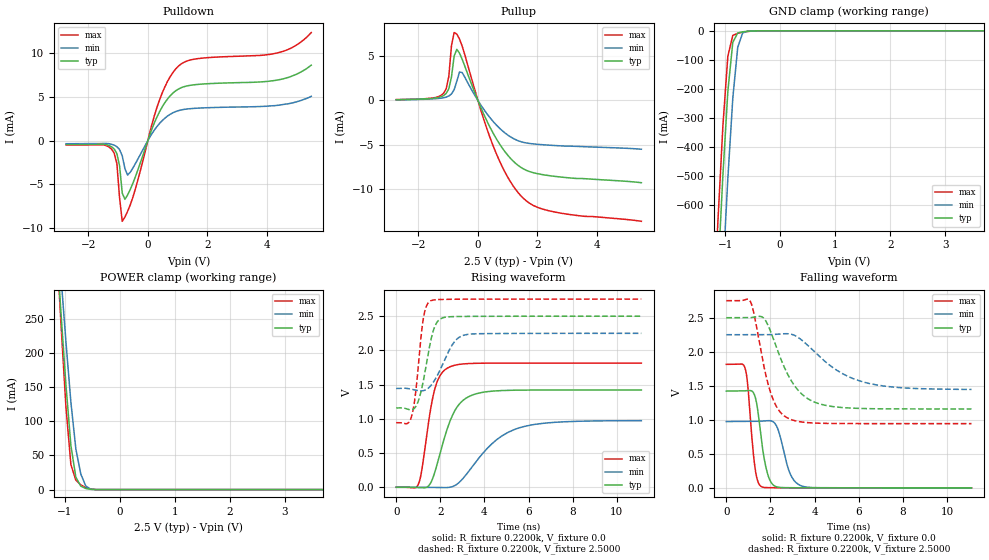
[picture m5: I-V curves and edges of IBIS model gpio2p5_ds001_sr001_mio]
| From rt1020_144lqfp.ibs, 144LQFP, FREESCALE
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[Model] gpio2p5_ds001_sr001_mio
|   Model gpio2p5_ds001_sr001_mio
| This model was characterised for following simulation conditions:
| External (pad) voltage:
|   - Typ: 2.5V,   - Min: 2.25V,   - Max: 2.75V
| Library cells for typ/min/max conditions are connected as defined below:
|  pad - External Pad
|  ipp_do - Core Input
|  ipp_obe - Output Buffer Enable
|  esd_boost - ovdd
|  ipp_dse0 - vddi
|  ipp_dse1 - vssi
|  ipp_dse2 - vssi
|  ipp_fsel0 - vddi
|  ipp_fsel1 - vssi
|  ipp_ina - ipp_ina
|  ipp_ind - ipp_ind
|  ipp_pwr_stable - vddi
|  ipp_sre - vssi
|  ovdd - ovdd
|  ovss - ovss
|  vddi - vddi
|  vssi - vssi
| All other pins connected to ground
Model_type I/O
Polarity   Non-Inverting
Enable   Active-High
Vinl =   0.7500V
Vinh =   1.7500V
Vmeas =  1.2500V
Cref =   0.0F
Rref =   0.2200k
Vref =   1.2500V
C_comp   1.2356pF   1.1994pF   1.2834pF
|C_comp_pullup   0.6221pF   0.6388pF   0.6072pF
|C_comp_pulldown   0.5474pF   0.5787pF   0.5258pF
[Model Spec]
| variable   typ   min   max
Vinh   1.7500V   1.5750V   1.9250V
Vinl   0.7500V   0.6750V   0.8250V
S_overshoot_high   2.5000V   2.2500V   2.7500V
S_overshoot_low   0.0V   0.0V   0.0V
Vmeas   1.2500V   1.1250V   1.3750V
Vref   1.2500V   1.1250V   1.3750V
Cref   0.0F   0.0F   0.0F
Rref   0.2200k   0.2200k   0.2200k
[Temperature Range]   25.0000   0.1050k   -20.0000
[Voltage Range]   2.5000V   2.2500V   2.7500V
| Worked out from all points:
|   slope of the pulldown table from 0 to 0.375 V, typ, clamps not added: 118 ohm
|   slope of the pullup table from 0 to 0.375 V, typ, clamps not added: 134 ohm
|   GND clamp passes 1 mA (typ) near -0.54 V on its own axis
|   POWER clamp passes 1 mA (typ) near -0.57 V on its own axis
|   rising waveform, R_fixture 0.2200k, V_fixture 0.0: 20-80 % time 882ps typ, 1.74ns min, 549ps max; typ from 0 V to 1.42 V
|   rising waveform, R_fixture 0.2200k, V_fixture 2.5000: 20-80 % time 484ps typ, 739ps min, 343ps max; typ from 1.16 V to 2.5 V
|   falling waveform, R_fixture 0.2200k, V_fixture 0.0: 20-80 % time 382ps typ, 492ps min, 286ps max; typ from 1.42 V to 0 V
|   falling waveform, R_fixture 0.2200k, V_fixture 2.5000: 20-80 % time 1.19ns typ, 2.03ns min, 756ps max; typ from 2.5 V to 1.16 V
[Pulldown]
|Voltage   I(typ)   I(min)   I(max)
-2.75V    -437uA     -349uA     -488uA
-1.22V    -696uA     -410uA     -955uA
-1.04V    -1.485mA   -688.7uA   -2.63mA
-950mV    -2.87mA    -1.013mA   -6.54mA
-860mV    -5.981mA   -1.728mA   -9.203mA
-770mV    -6.697mA   -3.198mA   -8.717mA
-680mV    -6.194mA   -3.924mA   -8.067mA
400mV     3.337mA    1.986mA    4.698mA
1.03V     5.893mA    3.429mA    8.508mA
1.66V     6.415mA    3.709mA    9.354mA
4.36V     6.92mA     4.03mA     10.01mA
5.5V      8.62mA     5.06mA     12.34mA
[Pullup]
|Voltage   I(typ)   I(min)   I(max)
-2.75V    90uA       80uA       100uA
-1.16V    543uA      304uA      797uA
-980mV    1.318mA    507uA      2.697mA
-890mV    2.653mA    742uA      6.183mA
-800mV    5.023mA    1.217mA    7.66mA
-710mV    5.768mA    2.181mA    7.493mA
-620mV    5.336mA    3.213mA    6.929mA
-530mV    4.654mA    3.148mA    6.127mA
550mV     -3.913mA   -2.508mA   -5.429mA
1.45V     -7.548mA   -4.649mA   -10.76mA
2.53V     -8.531mA   -5.066mA   -12.54mA
5.5V      -9.27mA    -5.494mA   -13.62mA
[GND_clamp]
|Voltage   I(typ)   I(min)   I(max)
-2.75V    -7.488A    -7.708A    -7.379A
-1.22V    -1.193A    -1.537A    -1.012A
-1.13V    -835.6mA   -1.18A     -654.7mA
-1.04V    -497.8mA   -833mA     -328mA
-950mV    -208.9mA   -508.7mA   -87.54mA
-860mV    -39.89mA   -232.5mA   -15.89mA
-770mV    -7.264mA   -56.44mA   -8.363mA
-680mV    -3.422mA   -7.048mA   -4.851mA
-590mV    -1.552mA   -1.455mA   -2.251mA
-500mV    -482.7uA   -438.2uA   -698.4uA
5.5V      0A         0A         0A
[POWER_clamp]
|Voltage   I(typ)   I(min)   I(max)
-2.75V    2.386A     2.288A     2.687A
-1.16V    368.2mA    410.8mA    372.9mA
-1.07V    258.5mA    311.8mA    242.5mA
-980mV    153.1mA    216.2mA    121.1mA
-890mV    64.5mA     128mA      36.56mA
-800mV    18.16mA    59.6mA     13.82mA
-710mV    5.012mA    22.76mA    6.935mA
-620mV    1.706mA    5.315mA    2.959mA
-530mV    383.1uA    636.8uA    795.1uA
-440mV    42.36uA    66.97uA    84.45uA
5.5V      0A         0A         0A
[Ramp]
| variable   typ   min   max
dV/dt_r  0.8533/0.8819n   0.5843/1.7431n   1.0888/0.5485n
dV/dt_f  0.8044/1.1876n   0.4823/2.0251n   1.0836/0.7560n
R_load = 0.2200k
[Rising Waveform]
R_fixture= 0.2200k
V_fixture= 0.0
V_fixture_min= 0.0
V_fixture_max= 0.0
|time   V(typ)   V(min)   V(max)
0s        3.706nV    14.41nV    11.69nV
1.008ns   -4.347mV   158.2uV    47.25mV
1.173ns   -6.462mV   -321.7uV   276.6mV
1.451ns   15.85mV    -1.638mV   917.6mV
1.749ns   219.5mV    -3.211mV   1.437V
2.382ns   918.7mV    -2.222mV   1.753V
3.354ns   1.335V     261.5mV    1.81V
4.533ns   1.409V     690.4mV    1.815V
5.569ns   1.42V      868.3mV    1.815V
11.11ns   1.422V     973.9mV    1.815V
[Rising Waveform]
R_fixture= 0.2200k
V_fixture= 2.5000
V_fixture_min= 2.2500
V_fixture_max= 2.7500
|time   V(typ)   V(min)   V(max)
0s        1.159V     1.444V     944mV
497.9ps   1.143V     1.446V     931.8mV
697.4ps   1.133V     1.434V     1.037V
880.3ps   1.178V     1.419V     1.38V
1.225ns   1.547V     1.412V     2.457V
1.549ns   2.118V     1.478V     2.723V
1.964ns   2.453V     1.699V     2.744V
2.584ns   2.494V     2.103V     2.748V
3.094ns   2.497V     2.225V     2.749V
11.11ns   2.5V       2.25V      2.75V
[Falling Waveform]
R_fixture= 0.2200k
V_fixture= 0.0
V_fixture_min= 0.0
V_fixture_max= 0.0
|time   V(typ)   V(min)   V(max)
0s        1.422V     974.5mV    1.815V
851.4ps   1.426V     976.8mV    1.756V
975.2ps   1.429V     977.1mV    1.493V
1.297ns   1.347V     977.7mV    301.8mV
1.587ns   715.4mV    980.4mV    18.61mV
1.83ns    252mV      986.4mV    3.768mV
2.091ns   52.62mV    976.7mV    2.188mV
2.908ns   2.078mV    196.6mV    562.5uV
3.441ns   1.134mV    24.83mV    215.8uV
11.11ns   209.4nV    8.599uV    -594.1nV
[Falling Waveform]
R_fixture= 0.2200k
V_fixture= 2.5000
V_fixture_min= 2.2500
V_fixture_max= 2.7500
|time   V(typ)   V(min)   V(max)
0s        2.5V       2.25V      2.75V
1.092ns   2.501V     2.25V      2.736V
1.261ns   2.51V      2.25V      2.546V
1.657ns   2.505V     2.25V      1.858V
2.041ns   2.269V     2.251V     1.366V
2.425ns   1.931V     2.261V     1.12V
2.823ns   1.642V     2.264V     1.018V
3.883ns   1.276V     2.035V     954.1mV
5.975ns   1.168V     1.578V     944.1mV
11.11ns   1.159V     1.446V     944mV
